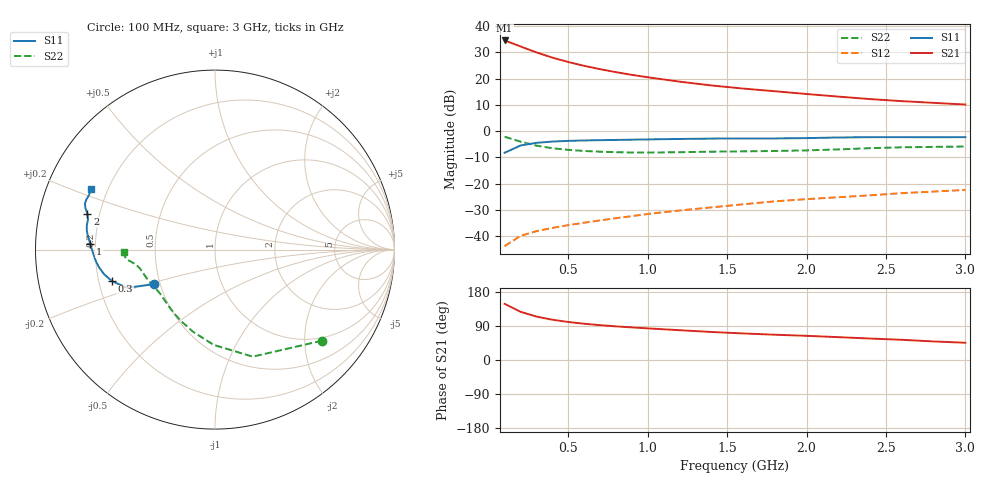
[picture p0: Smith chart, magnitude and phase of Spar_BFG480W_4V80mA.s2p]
! Filename: 480BFG480.001
! Title: BFG480W
! Bias: Vce=4V; Ic=80mA
! Company: NXP Semiconductors NL
! User: Quality&Reliability T&D
! Measure time: 10 Nov 1999 / 12:03:35
#  MHz  S  MA  R 50
! Freq  S11  S21  S12  S22  :
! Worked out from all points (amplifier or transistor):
!   20 points, 100 MHz to 3 GHz, reference 50 ohm
!   highest |S21| = 34.5 dB at 100 MHz (marker M1)
!   |S21| within 3 dB of that: start of sweep to 232.2 MHz
!   unconditionally stable (mu >= 1): 797.3 MHz to end of sweep
!   at 400 MHz: K = 0.76, MSG = 32.4 dB, |S12| = -36.8 dB
!   at 1.2 GHz: K = 1.07, MAG = 22.9 dB, |S12| = -30.2 dB
!   at 3 GHz: K = 1.05, MAG = 14.9 dB, |S12| = -22.3 dB
!   S11 on the Smith chart (normalised r, x): 100 MHz: 0.47, -0.21; 300 MHz: 0.26, -0.14; 1 GHz: 0.18, +0.02; 2 GHz: 0.15, +0.13; 3 GHz: 0.14, +0.23
100  0.3883 -150.3  53 148.2  0.006509 68.5  0.7832 -40.4
200  0.5334 -156.5  40.82 127.2  0.01023 59.3  0.6323 -70.6
300  0.5999 -162.9  31.41 114.7  0.01255 57.6  0.5309 -90.8
400  0.6335 -167.6  25.03 106.3  0.01447 58.7  0.4737 -105.0
500  0.6531 -171.2  20.65 100.3  0.01632 60.6  0.4407 -115.4
600  0.6655 -174.1  17.46 95.7  0.01817 62.5  0.4205 -123.2
700  0.6739 -176.6  15.09 92.0  0.02012 64.7  0.4071 -129.3
800  0.6811 -178.8  13.25 88.8  0.02217 66.5  0.3983 -134.4
900  0.6889 179.2  11.77 86.1  0.0242 68.4  0.3934 -138.8
1000  0.6961 177.3  10.59 83.5  0.02661 69.6  0.3923 -142.7
1200  0.7108 174.2  8.742 78.7  0.03101 71.6  0.3979 -149.1
1400  0.7216 171.8  7.404 74.0  0.03553 72.7  0.4071 -153.9
1600  0.7269 169.4  6.458 70.1  0.04067 73.8  0.4131 -157.5
1800  0.7273 166.7  5.743 66.7  0.0463 74.5  0.4199 -161.3
2000  0.7377 164.4  5.084 63.8  0.05101 75.4  0.4307 -165.7
2200  0.7579 162.3  4.539 60.3  0.05542 75.3  0.45 -169.5
2400  0.7686 160.5  4.071 56.6  0.06025 74.9  0.4744 -172.0
2600  0.7691 158.8  3.722 53.3  0.06631 74.3  0.4933 -173.5
2800  0.7649 156.6  3.452 48.9  0.07105 73.0  0.5024 -175.3
3000  0.77 153.9  3.206 45.5  0.07638 72.3  0.5098 -178.2
